(* Logix 5000 AddOnInstructionDefinition export Banner_QS18COD_PD_v4; software revision 33.00 *)

TYPE Banner_QS18COD_PDIO_v4 :   // Process Data for a QS18COD sensors.
STRUCT
   Output_State : SINT;   // 0 = Inactive, 1 = Active
   Health_Signal : SINT;   // 0 = Marginal or Worse, 1 = Healthy
   PDI_DT : SINT[2];
END_STRUCT
END_TYPE

ADD_ON_INSTRUCTION Banner_QS18COD_PD_v4   (* revision 4.0, vendor Banner Engineering *)
// Take raw process data and convert it to usable values.
VAR_IN_OUT
   Process_Data : Banner_QS18COD_PDIO_v4; {required}
END_VAR
VAR_INPUT
   Byte_Swap : BOOL; {required}
END_VAR
VAR
   Temp_Byte : SINT[4]; {access None}
END_VAR

ROUTINE Logic   (* ladder *)
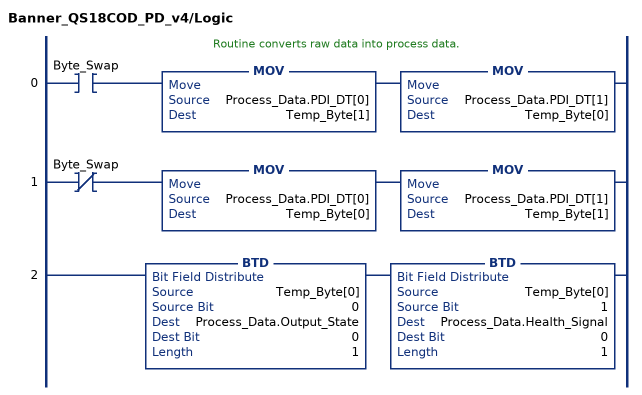
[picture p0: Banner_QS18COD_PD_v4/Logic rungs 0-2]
   // Routine converts raw data into process data.
   0: XIC(Byte_Swap)MOV(Process_Data.PDI_DT[0],Temp_Byte[1])MOV(Process_Data.PDI_DT[1],Temp_Byte[0]);
   1: XIO(Byte_Swap)MOV(Process_Data.PDI_DT[0],Temp_Byte[0])MOV(Process_Data.PDI_DT[1],Temp_Byte[1]);
   2: BTD(Temp_Byte[0],0,Process_Data.Output_State,0,1)BTD(Temp_Byte[0],1,Process_Data.Health_Signal,0,1);
END_ROUTINE
END_ADD_ON_INSTRUCTION
